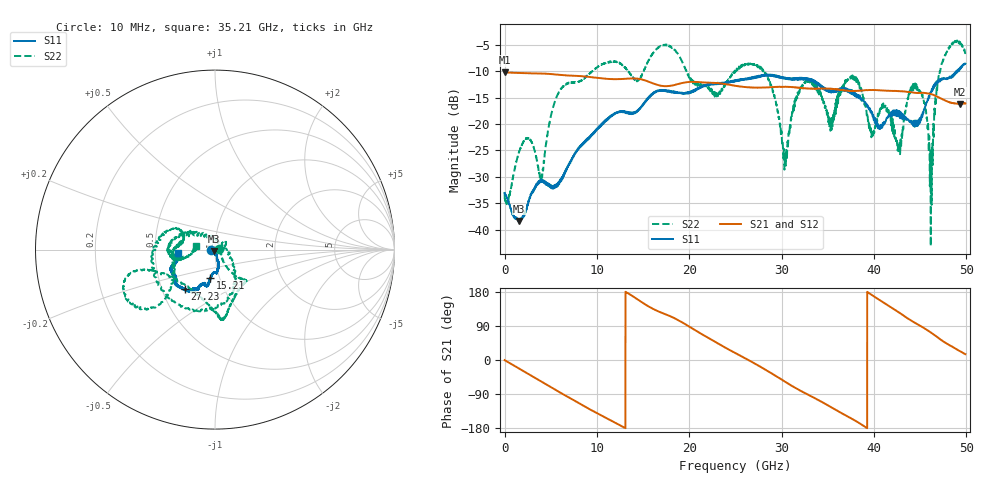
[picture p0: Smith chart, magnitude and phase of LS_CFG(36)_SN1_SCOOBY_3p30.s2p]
!Keysight Technologies,N5245B,MY58422026,A.13.80.08
!Date: Thursday, March 19, 2020 23:38:05
!Correction: S11(Full 2 Port(1,2))
!S21(Full 2 Port(1,2))
!S12(Full 2 Port(1,2))
!S22(Full 2 Port(1,2))
!S2P File: Measurements: S11, S21, S12, S22:
# Hz S DB R 50.0
!freq dBS11 angS11 dBS21 angS21 dBS12 angS12 dBS22 angS22
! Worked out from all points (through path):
!   4991 points, 10 MHz to 49.91 GHz, reference 50 ohm
!   highest |S21| = -10.21 dB at 10 MHz (marker M1); lowest = -16.2 dB at 49.34 GHz (marker M2)
!   group delay of S21, straight-line fit = 38.7 ps
!   lowest |S11| = -38.4 dB at 1.52 GHz (marker M3), VSWR 1.02, Z = 49.3 - j0.98 ohm
!   |S11| at or under -10 dB: start of sweep to 48.9 GHz; 48.92248 GHz to 49.00115 GHz (78.67 MHz wide, 0.161 % of centre); 49.06289 GHz to 49.09773 GHz (34.85 MHz wide, 0.071 % of centre)
!   |S22| runs from -43.1 to -4.2 dB; largest |S21 - S12| = 0.0028
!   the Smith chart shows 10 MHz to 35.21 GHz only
!   S11 on the Smith chart (normalised r, x): 10 MHz: 0.96, -0.01; 15.21 GHz: 0.90, -0.29; 27.23 GHz: 0.66, -0.31; 35.21 GHz: 0.66, -0.03
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1e7  -33.08 -172.8  -10.21 -0.3  -10.20 -0.3  -32.86 2.4
1.52e9  -38.37 -124.6  -10.30 -21.8  -10.29 -21.8  -25.62 14.2
3.96e9  -30.83 -79.3  -10.42 -56.4  -10.42 -56.3  -30.61 -3.8
5.64e9  -31.65 -81.1  -10.62 -80.7  -10.61 -80.7  -14.85 -51.8
8.33e9  -24.18 -76.6  -10.93 -117.7  -10.92 -117.6  -11.71 -58.9
1.521e10  -15.93 -99.6  -11.73 147.1  -11.72 147.1  -9.40 -158.7
1.665e10  -13.74 -102.4  -12.61 128.4  -12.61 128.5  -5.50 -160.8
2.288e10  -12.44 -113.6  -12.21 47.2  -12.21 47.3  -14.73 163.5
2.496e10  -11.88 -119.0  -12.71 18.8  -12.70 19.0  -10.13 170.0
2.723e10  -11.25 -127.3  -13.10 -11.2  -13.11 -11.1  -8.92 -114.3
3.038e10  -11.33 -144.3  -12.95 -57.3  -12.94 -57.1  -26.00 44.5
3.328e10  -11.68 -159.2  -13.28 -96.9  -13.28 -96.6  -11.88 -173.3
3.521e10  -13.64 -174.5  -13.31 -122.2  -13.25 -121.8  -19.35 168.6
3.758e10  -14.24 169.3  -13.72 -154.8  -13.65 -154.9  -11.05 155.4
3.981e10  -17.77 166.4  -13.55 171.0  -13.54 170.9  -21.72 -76.8
4.16e10  -18.33 104.4  -13.70 143.3  -13.72 143.2  -17.72 53.0
4.274e10  -18.42 95.9  -13.75 125.0  -13.78 124.9  -24.78 4.8
4.492e10  -19.20 34.3  -14.09 92.0  -14.11 91.9  -13.53 11.2
4.616e10  -13.91 9.5  -14.30 72.8  -14.32 72.8  -43.13 -40.2
4.723e10  -11.47 9.0  -15.12 53.9  -15.13 54.0  -9.37 -86.9
4.934e10  -9.56 -17.6  -16.17 23.0  -16.19 23.2  -4.45 -33.8
4.991e10  -8.55 -15.4  -16.07 15.3  -16.09 15.2  -6.50 -22.4
